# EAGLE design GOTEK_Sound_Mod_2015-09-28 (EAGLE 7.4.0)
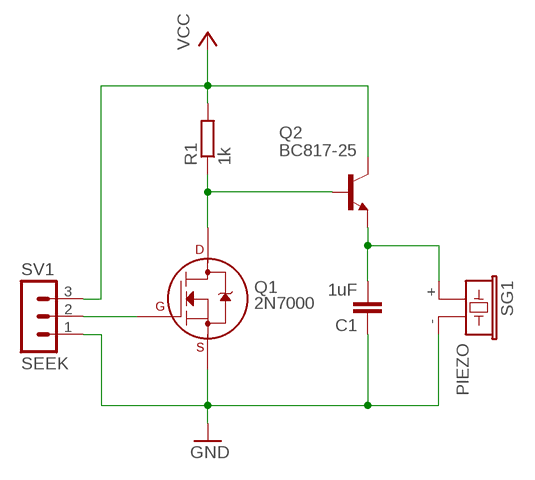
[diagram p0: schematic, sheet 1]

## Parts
C1  1uF  C-EUC0805  [C0805]
Q1  2N7000  2N7000_SOT23  [SOT-23]
Q2  BC817-25  BC817-25SMD  [SOT23-BEC]
R1  1k  R-EU_R0805  [R0805]
SG1  PIEZO  F/CM12P  [F/CM12P]
SV1  SEEK  MA03-1  [MA03-1]

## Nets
GND [power]: C1.1 Q1.2(S) SG1.- SV1.1
N$1: Q1.3(D) Q2.B R1.1
N$2: C1.2 Q2.E SG1.+
N$5: Q1.1(G) SV1.2
VCC [power]: Q2.C R1.2 SV1.3

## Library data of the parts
C1 = rcl:C-EU: CAPACITOR, European symbol
Q1 = transistors2:2N700*: 2N7000, 2N7002, NDS7002A N-channel enhancement mode MOSFET
Q2 = transistor-npn:BC817*: NPN Transistor
R1 = rcl:R-EU_: RESISTOR, European symbol
SG1 = buzzer:F/CM12P: BUZZER; OC_FARNELL: unknown; OC_NEWARK: unknown
SV1 = con-lstb:MA03-1: PIN HEADER; OC_FARNELL: unknown; OC_NEWARK: unknown

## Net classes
0 default: width 0.406 mm, drill 0.508 mm
1 power: width 0.813 mm, drill 0.762 mm, clearance 0.254 mm

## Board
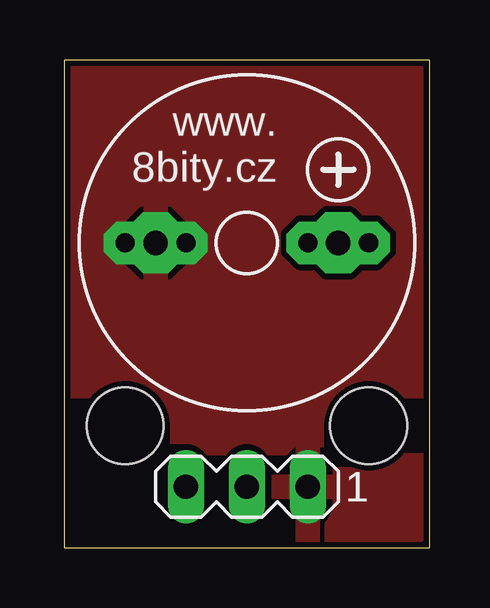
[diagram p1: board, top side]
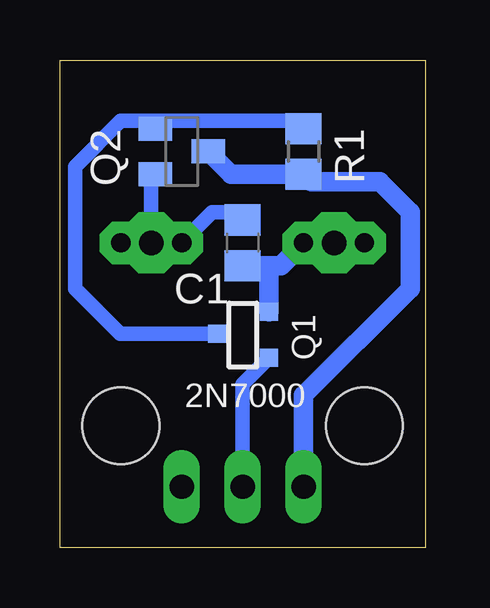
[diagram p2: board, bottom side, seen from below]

Size 15.24 x 20.32 mm. Coordinates in mm from the lower left corner, seen from the top.
Outline: 0,0 15.24,0 15.24,20.32 0,20.32 0,0
Copper layers (1*16): Top 0.035mm / dielectric 1.5mm / Bottom 0.035mm
Design rules "SeeedStudio_2layer_DRU_no_angle_20140221 *": minimum track width 6mil, minimum drill 12mil, track to track 6mil, track to pad 6mil, pad to pad 6mil, via to via 6mil, smd to smd 0mil, copper to edge 10mil, drill to drill 10mil, minimum pad ring 10mil, minimum via ring 6mil, stop-mask expansion 2mil, vias tented up to drill 100mil, thermal gap 10mil
Holes 3.2 mm at 2.54,5.08 12.7,5.08

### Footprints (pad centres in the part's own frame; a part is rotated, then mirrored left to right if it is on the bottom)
C0805 = smd 1.3 x 1.5: 1 -0.95,0; 2 0.95,0
SOT-23 = smd 0.762 x 0.762: 1 -0.979,-1.101; 2 0.94,-1.101; 3 0.025,1.067
SOT23-BEC = smd 1 x 1.4: B -0.95,-1.1; C 0,1.1; E 0.95,-1.1
R0805 = smd 1.3 x 1.5: 1 -0.95,0; 2 0.95,0
F/CM12P = drill 1.016 pad 2.54 octagon: + 3.81,0; - -3.81,0
MA03-1 = drill 1.016 long: 1 -2.54,0; 2 0,0; 3 2.54,0

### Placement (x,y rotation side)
C1  7.62,12.7 90 bottom
Q1  7.62,8.89 90 bottom
Q2  10.16,16.51 270 bottom
R1  5.08,16.51 270 bottom
SG1  7.62,12.7 0 top
SV1  7.62,2.54 180 top

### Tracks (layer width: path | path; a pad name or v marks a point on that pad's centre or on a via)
GND  (via drill 0.8 pad 1.78)
  Bottom 0.813: C1.1 6.35,11.75 | 6.35,11.75 6.03,11.75 v5.08,12.7 | Q1.2 6.52,11.58 6.35,11.75
  other vias: 2.54,12.7
  pour Top: 0.64,0.64 14.61,0.64 14.61,19.68 0.64,19.68
N$1
  Bottom 0.61: Q1.3 12.72,8.91 14.61,10.79 14.61,15.88 12.7,17.78 11.43,17.78 | 11.43,17.78 5.4,17.78 R1.1 | Q2.B 11.26,17.61 11.43,17.78
N$2  (via drill 0.8 pad 1.78)
  Bottom 0.61: SG1.+ 11.43,15.39 Q2.E | SG1.+ v10.16,12.7 8.89,13.97 7.94,13.97 C1.2 | v12.7,12.7 SG1.+
N$5
  Bottom 0.61: SV1.2 7.62,6.81 Q1.1
VCC
  Bottom 0.813: SV1.3 5.08,6.35 0.64,10.79 0.64,13.97 1.91,15.24 4.76,15.24 R1.2 8.11,15.56 Q2.C

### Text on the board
tPlace: www. / 8bity.cz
